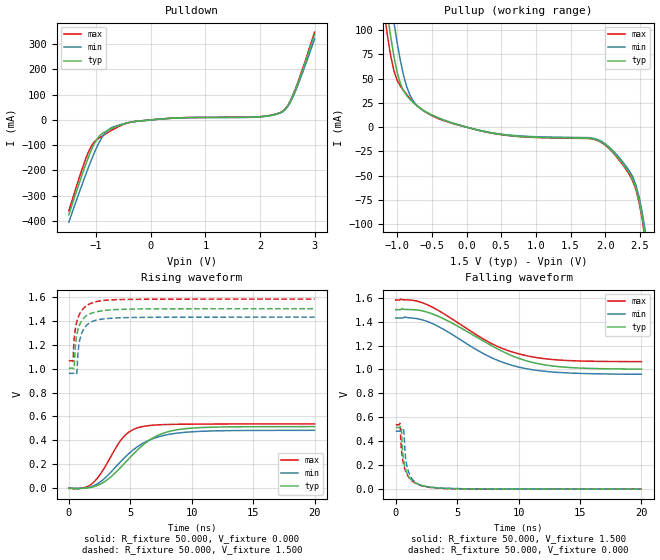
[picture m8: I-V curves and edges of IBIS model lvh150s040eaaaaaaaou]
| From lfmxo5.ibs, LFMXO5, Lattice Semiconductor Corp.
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[Model] lvh150s040eaaaaaaaou
Model_type Output
Polarity   Non-Inverting
Enable   Active-High
Vmeas =  0.750V
Cref =  0.0F
Rref =  1.000M
Vref =  0.0V
C_comp   5.000pF   4.000pF   5.500pF
[Temperature Range]   25.000   0.125k   -40.000
[Voltage Range]   1.500V   1.430V   1.580V
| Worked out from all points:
|   slope of the pulldown table from 0 to 0.225 V, typ, clamps not added: 52.2 ohm
|   slope of the pullup table from 0 to 0.225 V, typ, clamps not added: 56 ohm
|   rising waveform, R_fixture 50.000, V_fixture 0.000: 20-80 % time 3.21ns typ, 3.19ns min, 1.97ns max; typ from 0 V to 0.515 V
|   rising waveform, R_fixture 50.000, V_fixture 1.500: 20-80 % time 568ps typ, 544ps min, 611ps max; typ from 1 V to 1.5 V
|   falling waveform, R_fixture 50.000, V_fixture 1.500: 20-80 % time 5.43ns typ, 4.98ns min, 5.14ns max; typ from 1.5 V to 1 V
|   falling waveform, R_fixture 50.000, V_fixture 0.000: 20-80 % time 559ps typ, 544ps min, 606ps max; typ from 0.515 V to 0 V
[Pulldown]
|Voltage   I(typ)   I(min)   I(max)
-1.5V     -375.9mA   -405mA     -360mA
-1.224V   -196.9mA   -236.1mA   -174.2mA
-1.086V   -118.5mA   -157.8mA   -102.9mA
-948mV    -65.35mA   -90.4mA    -72.03mA
-764mV    -39.35mA   -37.22mA   -47.13mA
-258mV    -5.508mA   -5.47mA    -5.083mA
1.95V     11.93mA    11.34mA    12.29mA
2.364V    27.86mA    26.47mA    28.7mA
2.502V    53.11mA    50.46mA    54.71mA
2.594V    91mA       86.4mA     93.7mA
2.732V    167.3mA    158.9mA    172.3mA
3V        337.8mA    320.9mA    347.9mA
[Pullup]
|Voltage   I(typ)   I(min)   I(max)
-1.5V     334.2mA    366.8mA    315.2mA
-1.186V   140.5mA    179.9mA    117.2mA
-1.14V    115.6mA    154.7mA    93.3mA
-1.048V   72.68mA    107.9mA    57.95mA
-956mV    44.92mA    68.74mA    42.37mA
-864mV    32.38mA    41.6mA     33.55mA
-588mV    15.88mA    15.55mA    15.32mA
424mV     -6.746mA   -6.408mA   -6.948mA
1.896V    -13.58mA   -12.9mA    -13.99mA
2.402V    -54.62mA   -51.89mA   -56.26mA
2.586V    -116.3mA   -110.5mA   -119.8mA
3V        -369.7mA   -351.2mA   -380.8mA
[Ramp]
| variable   typ   min   max
dV/dt_r   0.309/3.231n   0.291/3.213n   0.333/2.014n
dV/dt_f   0.298/5.467n   0.282/4.991n   0.322/5.158n
R_load = 50.000
[Rising Waveform]
R_fixture = 50.000
V_fixture = 0.000
V_fixture_min = 0.000
V_fixture_max = 0.000
|  time   V(typ)   V(min)   V(max)
0s        59.51uV    153uV      -399.5uV
1.227ns   828.9uV    1.67mV     4.556mV
1.946ns   11.53mV    19.1mV     43.83mV
3.051ns   65.77mV    96.28mV    197.4mV
4.381ns   192.5mV    240.4mV    421mV
4.989ns   258.3mV    299.4mV    476.5mV
5.83ns    343.5mV    363.6mV    511.8mV
7.435ns   450.2mV    434.1mV    530.7mV
9.441ns   497.5mV    467.6mV    535.5mV
20ns      515.5mV    484.4mV    538.2mV
[Rising Waveform]
R_fixture = 50.000
V_fixture = 1.500
V_fixture_min = 1.430
V_fixture_max = 1.580
|  time   V(typ)   V(min)   V(max)
0s        1.003V     960.1mV    1.065V
334ps     1.003V     960.2mV    1.064V
417ps     1V         960.4mV    1.221V
527ps     1.18V      959.1mV    1.326V
627ps     1.268V     955.1mV    1.38V
756ps     1.329V     1.141V     1.426V
837ps     1.355V     1.211V     1.447V
1.286ns   1.429V     1.342V     1.512V
2.116ns   1.471V     1.401V     1.556V
20ns      1.5V       1.43V      1.581V
[Falling Waveform]
R_fixture = 50.000
V_fixture = 1.500
V_fixture_min = 1.430
V_fixture_max = 1.580
|  time   V(typ)   V(min)   V(max)
0s        1.5V       1.43V      1.581V
727ps     1.502V     1.439V     1.582V
1.547ns   1.499V     1.427V     1.575V
3.031ns   1.462V     1.381V     1.518V
4.79ns    1.376V     1.28V      1.408V
7.583ns   1.212V     1.109V     1.228V
10.19ns   1.087V     1.016V     1.126V
11.63ns   1.047V     990.7mV    1.097V
13.55ns   1.021V     973.4mV    1.077V
20ns      1.003V     960.1mV    1.065V
[Falling Waveform]
R_fixture = 50.000
V_fixture = 0.000
V_fixture_min = 0.000
V_fixture_max = 0.000
|  time   V(typ)   V(min)   V(max)
0s        515.5mV    484.4mV    538.2mV
346ps     515mV      484.1mV    547.9mV
444ps     521.9mV    484.3mV    360.9mV
547ps     341.9mV    485.4mV    262.2mV
637ps     251mV      494.9mV    210.8mV
780ps     176.5mV    290.7mV    157.3mV
879ps     143.9mV    211.6mV    131.9mV
1.367ns   67.93mV    81.29mV    66.52mV
2.257ns   27.23mV    25.96mV    23.88mV
20ns      59.51uV    153uV      -399.5uV
